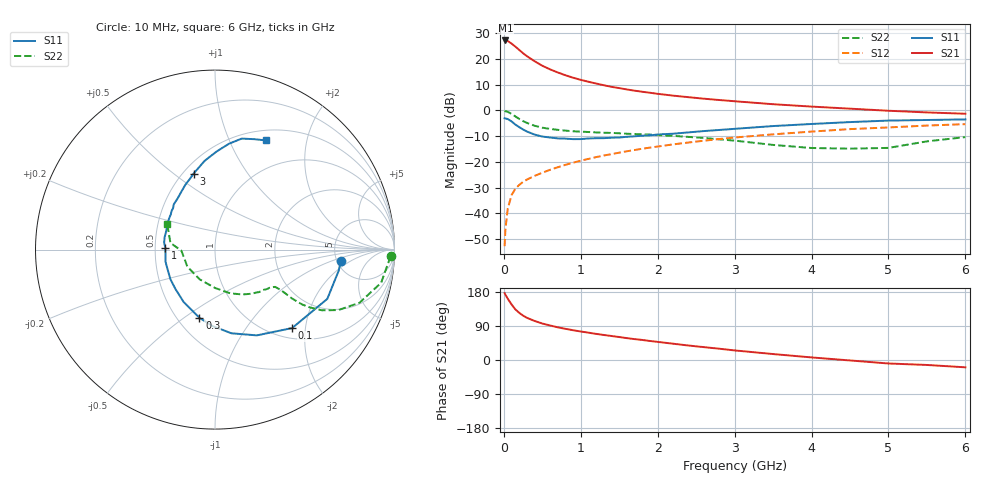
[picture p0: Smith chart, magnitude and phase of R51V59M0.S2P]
! SIEMENS Small Signal Semiconductors
! BFR183
! Si NPN RF Bipolar Junction Transistor in SOT23
! VCE = 1.5 V  IC = 9 mA
! Common Emitter S-Parameters:  May  1996
# GHz  S  MA  R  50
!  f  S11  S21  S12  S22
! GHz  MAG  ANG  MAG  ANG  MAG  ANG  MAG  ANG
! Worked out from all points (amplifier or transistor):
!   36 points, 10 MHz to 6 GHz, reference 50 ohm
!   highest |S21| = 27.2 dB at 20 MHz (marker M1)
!   |S21| within 3 dB of that: start of sweep to 173.3 MHz
!   unconditionally stable (mu >= 1): 776.7 MHz to 2.573 GHz
!   at 250 MHz: K = 0.60, MSG = 25.0 dB, |S12| = -27.7 dB
!   at 1.4 GHz: K = 1.06, MAG = 11.5 dB, |S12| = -17.0 dB
!   at 6 GHz: K = 0.91, MSG = 2.0 dB, |S12| = -5.3 dB
!   S11 on the Smith chart (normalised r, x): 10 MHz: 5.43, -1.32; 100 MHz: 1.21, -1.69; 300 MHz: 0.64, -0.57; 1 GHz: 0.57, +0.01; 3 GHz: 0.56, +0.59; 6 GHz: 0.62, +1.37
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0.01  0.7045 -5.0  22.95 176.5  0.0023 87.9  0.9795 -2.2
0.02  0.699 -9.7  22.98 172.4  0.0048 89.6  0.9671 -4.6
0.05  0.6833 -23.7  22.45 162.0  0.0122 78.7  0.944 -11.3
0.1  0.613 -45.5  20.03 146.7  0.0225 71.2  0.8577 -20.2
0.15  0.5317 -64.0  17.43 133.5  0.0302 65.4  0.7658 -26.1
0.2  0.4752 -78.9  15.04 124.4  0.0357 62.2  0.6846 -29.6
0.25  0.4269 -91.6  12.97 117.2  0.041 60.3  0.622 -31.3
0.3  0.3899 -102.8  11.37 111.3  0.0453 60.4  0.5741 -32.2
0.4  0.3399 -121.0  9.067 103.0  0.0535 60.4  0.5047 -32.4
0.5  0.311 -135.1  7.41 96.2  0.0617 61.5  0.4632 -31.9
0.6  0.2985 -146.2  6.313 91.1  0.0701 62.2  0.4381 -31.7
0.7  0.2865 -156.9  5.495 86.3  0.0787 63.0  0.4204 -31.6
0.8  0.2838 -166.7  4.843 82.3  0.0876 63.1  0.406 -31.7
1  0.2777 177.7  3.938 75.2  0.1054 63.5  0.3878 -32.5
1.1  0.2859 172.2  3.619 72.1  0.1145 63.4  0.3813 -33.6
1.6  0.3079 146.8  2.56 57.7  0.1611 61.1  0.353 -39.3
2.2  0.3532 126.1  1.943 43.0  0.219 56.3  0.3212 -49.8
3  0.4396 105.8  1.512 25.3  0.298 47.4  0.2594 -70.4
3.5  0.4977 96.7  1.324 15.7  0.3434 41.2  0.2139 -89.9
4.5  0.5948 82.5  1.085 -1.2  0.4344 28.4  0.181 -148.2
5.5  0.6531 70.4  0.917 -13.1  0.5089 16.4  0.251 171.5
6  0.6707 65.1  0.864 -19.3  0.5427 8.6  0.3037 151.4
